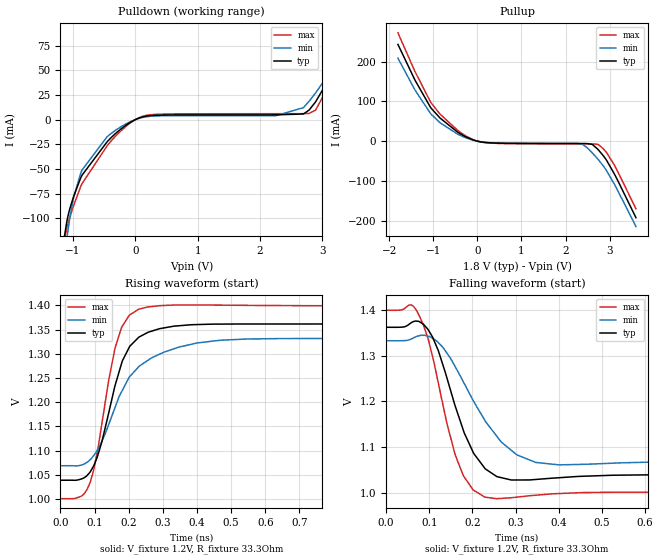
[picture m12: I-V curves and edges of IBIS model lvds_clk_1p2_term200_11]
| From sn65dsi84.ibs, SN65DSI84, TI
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|   Model
[Model]   lvds_clk_1p2_term200_11
Model_type   Output
Polarity   Non-Inverting
Vmeas = 1.2
Vref = 1.2
Cref = 1pF
Rref = 50
|   typ   min   max
C_comp   0.4797pF   0.3035pF   0.7186pF
[Voltage Range]   1.8   1.65   1.95
[Temperature Range]   27   125   -40
[Pullup Reference]   1.8   1.65   1.95
[Pulldown Reference]   -0   -0   -0
[Power Clamp Reference]   1.8   1.65   1.95
[GND Clamp Reference]   -0   -0   -0
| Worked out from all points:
|   slope of the pulldown table from 0 to 0.27 V, typ, clamps not added: 63.7 ohm
|   slope of the pullup table from 0 to 0.27 V, typ, clamps not added: 68 ohm
|   falling waveform, V_fixture 1.2V, R_fixture 33.3Ohm: 20-80 % time 68.7ps typ, 100ps min, 59.1ps max; typ from 1.36 V to 1.04 V
|   rising waveform, V_fixture 1.2V, R_fixture 33.3Ohm: 20-80 % time 74.8ps typ, 118ps min, 60ps max; typ from 1.04 V to 1.36 V
[Pulldown]
|   Voltage   I(typ)   I(min)   I(max)
-1.8V     -662.8mA   -697.9mA   -653.3mA
-1.141V   -120.2mA   -145.2mA   -123.4mA
-1.087V   -100mA     -116mA     -107.2mA
-990mV    -78.03mA   -79.28mA   -87.36mA
-855mV    -56.34mA   -51.07mA   -64.87mA
-450mV    -22.28mA   -17.17mA   -26.37mA
-190.8mV  -7.546mA   -5.748mA   -9.037mA
79.2mV    2.067mA    1.609mA    2.504mA
2.261V    4.896mA    4.121mA    6.046mA
2.698V    5.776mA    12.21mA    6.092mA
2.893V    18.05mA    27.07mA    9.678mA
3.595V    93.25mA    90.74mA    91.15mA
[Pullup]
|   Voltage   I(typ)   I(min)   I(max)
-1.8V     243.1mA    208.5mA    272.3mA
-1.417V   154mA      129mA      175.6mA
-1.049V   83.18mA    68.11mA    96.65mA
-450mV    22.93mA    17.9mA     27.39mA
-115.2mV  3.989mA    3.171mA    4.762mA
171mV     -3.141mA   -2.871mA   -3.537mA
2.38V     -5.94mA    -7.661mA   -6.963mA
2.606V    -8.382mA   -29.65mA   -7.096mA
2.747V    -22.49mA   -47.11mA   -8.852mA
2.903V    -43.97mA   -70.08mA   -25.25mA
3.141V    -90.1mA    -115.6mA   -67.62mA
3.595V    -192.4mA   -214.7mA   -170mA
[Ramp]
R_load = 33.3
|   typ   min   max
dV/dt_r   0.193674/7.47614e-11   0.15783/1.18301e-10   0.238941/6.00394e-11
dV/dt_f   0.193674/6.87202e-11   0.158234/1.00487e-10   0.238889/5.90689e-11
[Falling Waveform]
V_fixture = 1.2V
V_fixture_min = 1.2V
V_fixture_max = 1.2V
R_fixture = 33.3Ohm
C_fixture = 0F
|   Time   V(typ)   V(min)   V(max)
0s        1.362V     1.332V     1.399V
63.2ps    1.374V     1.338V     1.408V
97.17ps   1.357V     1.342V     1.337V
121ps     1.311V     1.328V     1.24V
160.1ps   1.19V      1.275V     1.083V
201.5ps   1.089V     1.202V     1.006V
228.6ps   1.053V     1.158V     990.3mV
266.8ps   1.033V     1.111V     987.5mV
346.7ps   1.029V     1.066V     994.4mV
1ns       1.039V     1.069V     1.001V
[Rising Waveform]
V_fixture = 1.2V
V_fixture_min = 1.2V
V_fixture_max = 1.2V
R_fixture = 33.3Ohm
C_fixture = 0F
|   Time   V(typ)   V(min)   V(max)
0s        1.039V     1.069V     1.001V
63.2ps    1.042V     1.071V     1.007V
87.21ps   1.056V     1.082V     1.035V
121ps     1.118V     1.119V     1.154V
160.1ps   1.235V     1.19V      1.313V
178.9ps   1.28V      1.222V     1.355V
228.6ps   1.334V     1.273V     1.392V
346.7ps   1.358V     1.314V     1.401V
467.7ps   1.361V     1.328V     1.401V
1ns       1.362V     1.332V     1.399V
